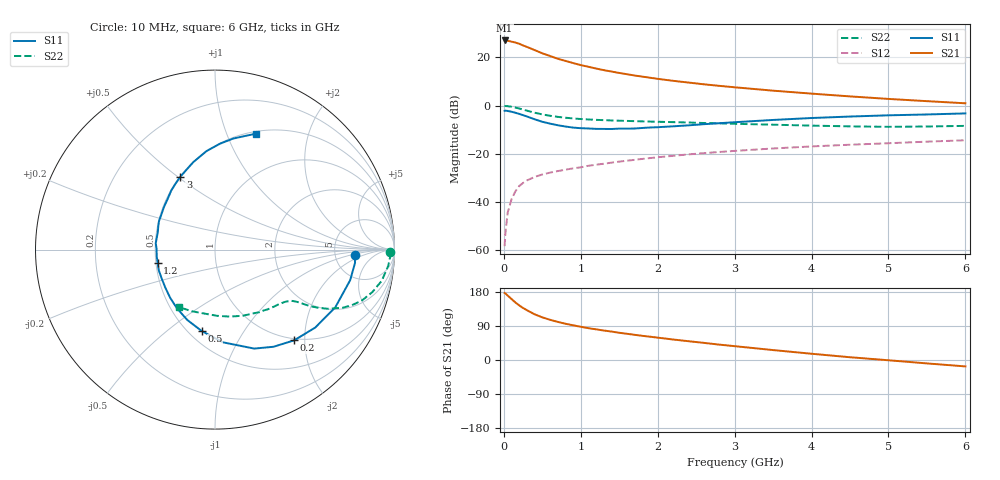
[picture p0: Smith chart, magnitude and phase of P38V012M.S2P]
! SIEMENS Small Signal Semiconductors
! BFP181
! Si NPN RF Bipolar Junction Transistor in SOT143
! VCE = 8 V  IC = 12 mA
! Common Emitter S-Parameters:  March  1996
# GHz  S  MA  R  50
!  f  S11  S21  S12  S22
! GHz  MAG  ANG  MAG  ANG  MAG  ANG  MAG  ANG
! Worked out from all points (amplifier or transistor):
!   36 points, 10 MHz to 6 GHz, reference 50 ohm
!   highest |S21| = 27.0 dB at 10 MHz (marker M1)
!   |S21| within 3 dB of that: start of sweep to 324.3 MHz
!   unconditionally stable (mu >= 1): 1.239 GHz to end of sweep
!   at 250 MHz: K = 0.33, MSG = 28.6 dB, |S12| = -32.1 dB
!   at 1.4 GHz: K = 1.04, MAG = 17.7 dB, |S12| = -23.7 dB
!   at 6 GHz: K = 1.02, MAG = 6.8 dB, |S12| = -14.4 dB
!   S11 on the Smith chart (normalised r, x): 10 MHz: 7.80, -1.29; 200 MHz: 0.97, -1.78; 500 MHz: 0.58, -0.67; 1.2 GHz: 0.51, -0.08; 3 GHz: 0.50, +0.51; 6 GHz: 0.52, +1.28
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0.01  0.7781 -2.4  22.47 176.9  0.0012 80.0  0.9762 -0.9
0.02  0.7838 -5.4  22.46 175.7  0.0022 79.0  0.9778 -2.0
0.05  0.772 -12.8  22.21 170.0  0.006 86.3  0.9693 -5.4
0.1  0.7433 -25.7  21.23 160.9  0.0113 75.5  0.9451 -10.6
0.15  0.7074 -37.9  20.35 151.9  0.0165 70.6  0.9082 -15.1
0.2  0.6709 -48.9  19.18 144.1  0.0213 67.0  0.8675 -19.0
0.25  0.6317 -59.0  17.7 137.2  0.0247 63.4  0.8235 -22.1
0.3  0.5931 -68.4  16.5 131.4  0.0278 60.0  0.7829 -24.4
0.4  0.5182 -85.2  14.19 120.6  0.0329 56.4  0.7095 -27.7
0.5  0.4595 -99.3  12.15 112.6  0.037 52.9  0.6544 -29.6
0.6  0.4214 -111.5  10.7 106.1  0.0404 52.3  0.6129 -30.8
0.7  0.3896 -123.0  9.374 100.6  0.0435 51.2  0.5818 -31.5
0.9  0.3486 -142.6  7.634 91.6  0.0496 50.7  0.5395 -32.6
1.1  0.3338 -159.8  6.378 84.0  0.0562 50.0  0.5132 -33.8
1.2  0.3276 -167.3  5.866 80.9  0.059 49.7  0.5047 -34.6
1.7  0.3335 162.7  4.206 66.5  0.0745 48.9  0.4737 -39.4
2.2  0.3701 140.3  3.263 54.1  0.0902 46.4  0.4519 -45.7
3  0.4502 115.3  2.394 36.5  0.1142 40.9  0.4175 -57.9
3.5  0.5018 104.0  2.036 26.2  0.1283 37.0  0.4 -67.1
4.5  0.5907 87.3  1.548 7.3  0.1535 28.9  0.3692 -88.2
5.5  0.6524 75.6  1.233 -9.0  0.1778 21.8  0.367 -110.6
6  0.6861 70.4  1.113 -16.9  0.1899 17.7  0.3781 -122.0
